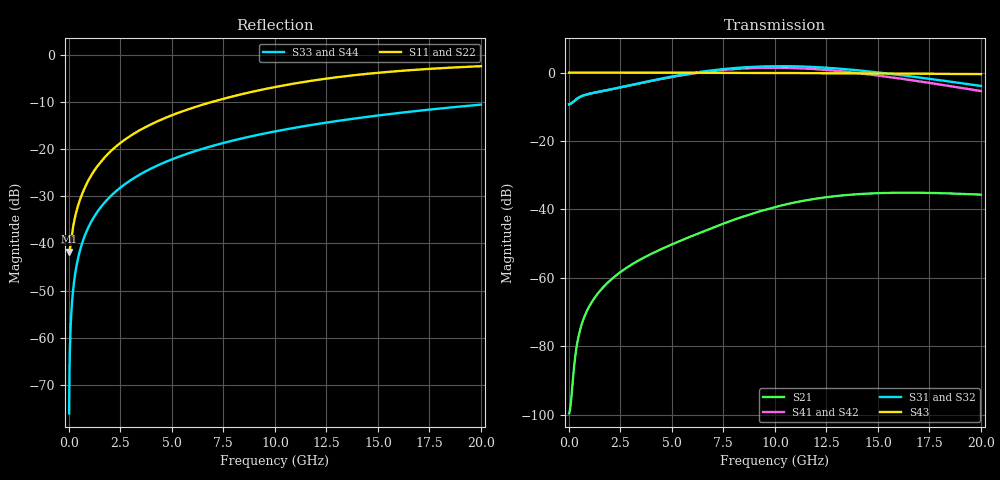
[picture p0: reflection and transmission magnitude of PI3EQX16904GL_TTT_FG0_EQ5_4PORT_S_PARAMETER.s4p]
! NPort=4 DATA=2000 NOISE=0 GROUPDELAY=0 COMPLEX_DATAFORMAT=POLAR
! NumOfBlock=1 NumOfParam=0
! .MODEL Smodel S TSTONEFILE=PI3EQX16904GL_TTT_FG0_EQ5_4PORT_S_PARAMETER.s4p TYPE=S
!  -- The above .MODEL line can be used for the S element in the netlist.
! The s parameter is extracted from the linear redriver, it is not bi-directional; only s(4,1)s(4,2) and s(3,1)s(3,2)
! should be the insertion loss
!Port definition:
!Port1 = input+
!Port2 = input-
!Port3 = output+
!Port4 = output-
# Hz S MA R  50
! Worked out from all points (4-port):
!   2000 points, 10 MHz to 20 GHz, reference 50 ohm
!   strongest paths, dB at 10 MHz, 5.01 GHz, 10.01 GHz, 15.01 GHz, 20 GHz:
!     S43: 0.0, 0.0, -0.1, -0.3, -0.4
!     S31: -9.2, -1.2, 1.9, 0.0, -3.9
!     S32: -9.2, -1.3, 1.7, -0.2, -4.2
!     S41: -9.2, -1.3, 1.4, -0.9, -5.4
!     S42: -9.2, -1.4, 1.2, -1.1, -5.7
!     S21: -99.6, -50.2, -39.3, -35.2, -35.7
!   lowest |S11| = -41.7 dB at 10 MHz (marker M1), VSWR 1.02, Z = 49.2 - j0.0603 ohm
!   |S11| at or under -10 dB: start of sweep to 6.888 GHz
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1e7  0.008182 -175.7  1.05e-05 7.7  0 0.0  0 0.0
     1.05e-05 7.7  0.008182 -175.7  0 0.0  0 0.0
     0.3452 0.5  0.3452 -179.5  0.0001571 -90.0  1 -0.0
     0.3452 -179.5  0.3452 0.4  1 -0.0  0.0001571 -90.0
6.2e8  0.03267 -112.4  0.0002097 114.7  0 0.0  0 0.0
       0.0002097 114.7  0.03268 -112.4  0 0.0  0 0.0
       0.4527 9.9  0.4524 -170.3  0.009738 -90.6  0.9999 -0.6
       0.4526 -171.2  0.4523 8.6  0.9999 -0.6  0.009738 -90.6
2.97e9  0.1382 -101.5  0.001518 103.1  0 0.0  0 0.0
        0.001516 103.1  0.1383 -101.5  0 0.0  0 0.0
        0.6538 -3.4  0.6498 175.8  0.0466 -92.8  0.9988 -2.7
        0.6509 171.3  0.6469 -9.5  0.9988 -2.7  0.0466 -92.8
6.3e9  0.2894 -105.4  0.004529 93.1  0 0.0  0 0.0
       0.004492 93.3  0.2893 -105.4  0 0.0  0 0.0
       1.016 -41.2  0.9974 137.8  0.09844 -95.9  0.9948 -5.6
       0.9954 127.6  0.9777 -53.4  0.9948 -5.6  0.09844 -95.9
9.89e9  0.4537 -112.5  0.01072 65.9  0 0.0  0 0.0
        0.01062 66.7  0.4533 -112.5  0 0.0  0 0.0
        1.239 -97.6  1.21 81.5  0.1534 -99.2  0.9872 -8.8
        1.181 65.1  1.153 -115.8  0.9872 -8.8  0.1534 -99.2
1.4e10  0.6184 -123.0  0.01682 19.8  0 0.0  0 0.0
        0.01671 21.1  0.618 -122.9  0 0.0  0 0.0
        1.081 -163.0  1.052 16.2  0.2144 -102.9  0.9749 -12.4
        0.9862 -6.6  0.9595 172.5  0.9749 -12.4  0.2144 -102.9
2e10  0.7648 -136.2  0.01647 -34.1  0 0.0  0 0.0
      0.01646 -32.1  0.7649 -136.1  0 0.0  0 0.0
      0.6381 118.5  0.6169 -62.2  0.2986 -108.1  0.9506 -17.4
      0.5373 -93.4  0.5195 85.8  0.9506 -17.4  0.2986 -108.1
